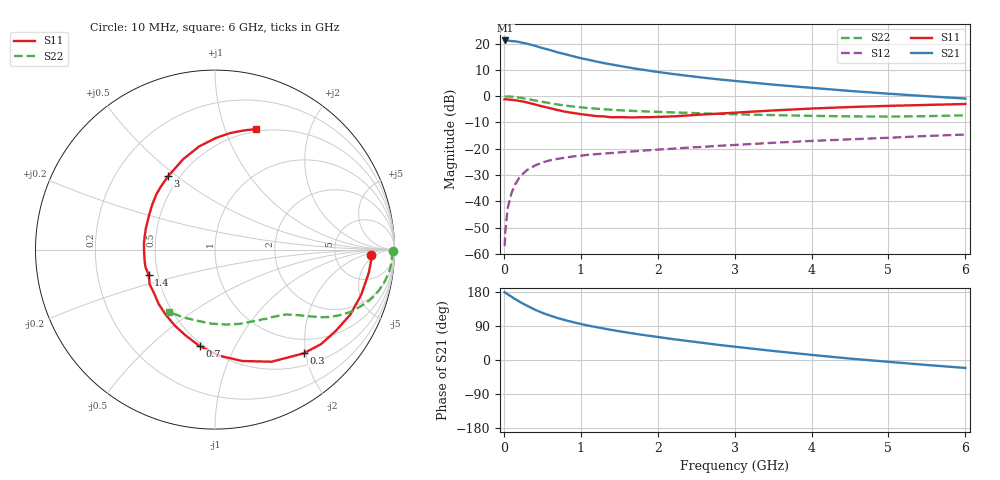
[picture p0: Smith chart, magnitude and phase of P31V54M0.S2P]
! SIEMENS Small Signal Semiconductors
! BFP181
! Si NPN RF Bipolar Junction Transistor in SOT143
! VCE = 1.5 V  IC = 4 mA
! Common Emitter S-Parameters:  March  1996
# GHz  S  MA  R  50
!  f  S11  S21  S12  S22
! GHz  MAG  ANG  MAG  ANG  MAG  ANG  MAG  ANG
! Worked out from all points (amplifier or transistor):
!   36 points, 10 MHz to 6 GHz, reference 50 ohm
!   highest |S21| = 21.2 dB at 20 MHz (marker M1)
!   |S21| within 3 dB of that: start of sweep to 515.7 MHz
!   unconditionally stable (mu >= 1): 1.718 GHz to end of sweep
!   at 250 MHz: K = 0.20, MSG = 24.9 dB, |S12| = -29.5 dB
!   at 1.4 GHz: K = 0.89, MSG = 16.8 dB, |S12| = -21.6 dB
!   at 6 GHz: K = 1.08, MAG = 5.1 dB, |S12| = -14.6 dB
!   S11 on the Smith chart (normalised r, x): 10 MHz: 14, -3; 300 MHz: 0.72, -1.96; 700 MHz: 0.48, -0.73; 1.4 GHz: 0.44, -0.15; 3 GHz: 0.43, +0.47; 6 GHz: 0.47, +1.29
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0.01  0.8698 -1.9  11.4 178.8  0.0014 86.5  0.991 -0.6
0.02  0.8725 -3.7  11.49 177.9  0.0027 89.4  0.9858 -1.4
0.05  0.8671 -8.4  11.45 173.4  0.0074 85.4  0.9874 -3.8
0.15  0.8365 -25.6  11.05 160.5  0.0214 75.6  0.9603 -11.0
0.2  0.8114 -33.9  10.73 154.4  0.028 72.2  0.9401 -14.2
0.25  0.7917 -41.7  10.3 148.6  0.0336 67.5  0.9145 -17.3
0.3  0.7601 -49.5  9.996 143.5  0.0392 63.9  0.8878 -19.9
0.4  0.6999 -63.2  9.146 133.1  0.0477 57.4  0.8327 -24.6
0.5  0.6387 -76.3  8.247 124.5  0.0546 52.4  0.7814 -28.0
0.6  0.5913 -87.8  7.548 117.2  0.0603 48.5  0.7356 -30.7
0.7  0.5442 -99.1  6.81 110.7  0.0642 45.4  0.6955 -32.8
0.8  0.5063 -108.7  6.285 104.9  0.0677 42.9  0.6621 -34.3
0.9  0.4793 -117.8  5.756 99.9  0.0714 40.9  0.6354 -35.7
1.1  0.4364 -136.0  4.927 90.6  0.0769 38.3  0.5935 -38.0
1.4  0.3959 -158.9  4.01 79.4  0.0829 35.7  0.5519 -41.1
1.8  0.3975 174.1  3.197 66.4  0.0921 34.1  0.5159 -45.3
2.2  0.4123 153.7  2.642 55.1  0.1003 32.9  0.4907 -50.2
3  0.4855 122.6  1.953 35.1  0.1179 29.8  0.4515 -62.2
3.5  0.5347 109.2  1.659 23.9  0.1298 27.6  0.4366 -71.3
4.5  0.6214 89.7  1.258 3.7  0.151 21.9  0.4131 -92.6
5.5  0.6819 76.6  0.998 -13.2  0.1749 16.9  0.4171 -115.3
6  0.7102 71.1  0.901 -21.0  0.1864 13.4  0.4314 -126.7
